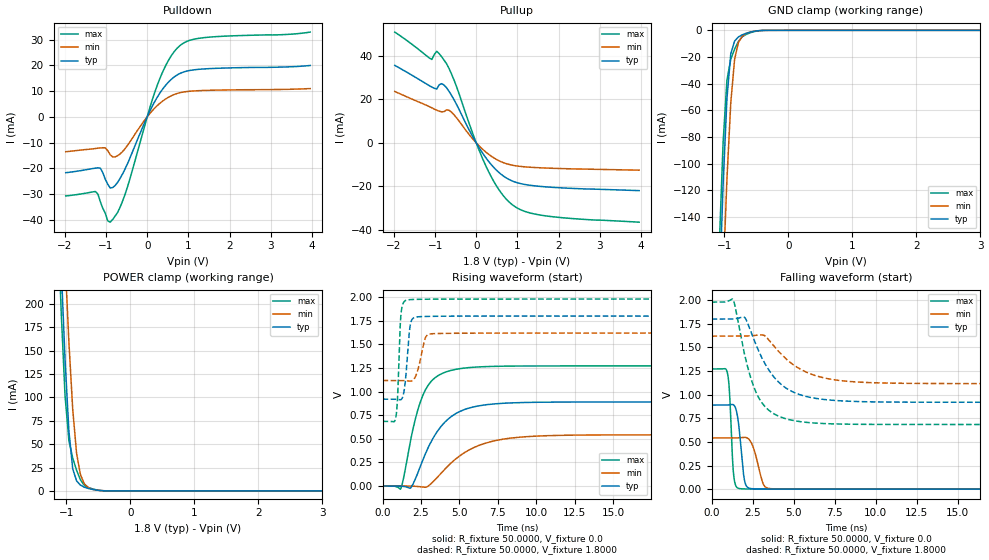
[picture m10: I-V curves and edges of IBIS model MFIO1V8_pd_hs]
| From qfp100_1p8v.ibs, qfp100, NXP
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[Model] MFIO1V8_pd_hs
|   Model MFIO1V8_pd_hs
| This model was characterised for following simulation conditions:
| External (pad) voltage:
|   - Typ: 1.8V,   - Min: 1.62V,   - Max: 1.98V
| Library cells for typ/min/max conditions are connected as defined below:
|  IO - External Pad
|  A - Core Input
|  EN - Output Buffer Enable
|  BOOST - vdde
|  EHS - vdd
|  ENZI - vdd
|  EPD - vdd
|  EPUN - vdd
|  ZI - NC
|  ZIF - NC
|  gnd - gnd
|  gnde - gnde
|  vdd - vdd
|  vdde - vdde
| All other pins connected to ground
Model_type I/O
Polarity   Non-Inverting
Enable   Active-Low
Vinl =   0.5400V
Vinh =   1.2600V
Vmeas =  0.9000V
Cref =   0.0F
Rref =   100.0000
Vref =   0.0V
C_comp   1.5958pF   1.5126pF   1.6704pF
|C_comp_pullup   0.7898pF   0.8219pF   0.7460pF
|C_comp_pulldown   0.5931pF   0.6315pF   0.5575pF
[Model Spec]
| variable   typ   min   max
Vinh   0.5400V   0.4860V   0.5940V
Vinl   1.2600V   1.1340V   1.3860V
Vmeas   0.9000V   0.8100V   0.9900V
[Temperature Range]   25.0000   0.1250k   -40.0000
[Voltage Range]   1.8000V   1.6200V   1.9800V
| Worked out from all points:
|   slope of the pulldown table from 0 to 0.27 V, typ, clamps not added: 32.6 ohm
|   slope of the pullup table from 0 to 0.27 V, typ, clamps not added: 34.8 ohm
|   GND clamp passes 1 mA (typ) near -0.56 V on its own axis
|   POWER clamp passes 1 mA (typ) near -0.54 V on its own axis
|   rising waveform, R_fixture 50.0000, V_fixture 0.0: 20-80 % time 1.9ns typ, 2.67ns min, 1.22ns max; typ from 0 V to 0.89 V
|   rising waveform, R_fixture 50.0000, V_fixture 1.8000: 20-80 % time 264ps typ, 419ps min, 177ps max; typ from 0.92 V to 1.8 V
|   falling waveform, R_fixture 50.0000, V_fixture 0.0: 20-80 % time 304ps typ, 487ps min, 201ps max; typ from 0.89 V to 0 V
|   falling waveform, R_fixture 50.0000, V_fixture 1.8000: 20-80 % time 1.84ns typ, 2.29ns min, 1.28ns max; typ from 1.8 V to 0.92 V
[Pulldown]
|Voltage   I(typ)   I(min)   I(max)
-1.98V    -21.74mA   -13.58mA   -30.76mA
-1.26V    -19.96mA   -12.33mA   -29.04mA
-1.14V    -19.96mA   -12.1mA    -33mA
-960mV    -26.19mA   -13.15mA   -40.44mA
-840mV    -27.51mA   -15.58mA   -39.92mA
-540mV    -20.34mA   -12.41mA   -30.2mA
60mV      2.086mA    1.197mA    3.341mA
300mV     9.043mA    5.145mA    14.58mA
540mV     13.88mA    7.813mA    22.59mA
840mV     17.16mA    9.517mA    28.23mA
1.44V     18.67mA    10.27mA    30.87mA
3.96V     19.95mA    10.98mA    32.93mA
[Pullup]
|Voltage   I(typ)   I(min)   I(max)
-1.98V    35.7mA     23.68mA    51.03mA
-1.08V    25.71mA    16.17mA    38.42mA
-960mV    24.81mA    15.04mA    42.18mA
-840mV    27.29mA    14.27mA    39.65mA
-720mV    25.36mA    15.21mA    36.42mA
-540mV    19.88mA    12.94mA    28.95mA
-60mV     2.001mA    1.263mA    3.041mA
240mV     -7.02mA    -4.333mA   -10.88mA
600mV     -14.41mA   -8.644mA   -22.88mA
900mV     -17.74mA   -10.36mA   -28.83mA
1.74V     -20.33mA   -11.62mA   -33.75mA
3.96V     -22mA      -12.58mA   -36.53mA
[GND_clamp]
|Voltage   I(typ)   I(min)   I(max)
-1.98V    -1.781A    -1.801A    -1.77A
-1.08V    -200.1mA   -270.2mA   -162.2mA
-1.02V    -116mA     -186.2mA   -84.49mA
-960mV    -51.26mA   -111.8mA   -37.36mA
-900mV    -17.65mA   -54.44mA   -21.7mA
-840mV    -8.02mA    -21.7mA    -14.08mA
-780mV    -4.924mA   -8.964mA   -8.313mA
-720mV    -3.338mA   -4.442mA   -4.753mA
-600mV    -1.403mA   -1.338mA   -1.896mA
-480mV    -330.4uA   -347.3uA   -423.3uA
-360mV    -26.82uA   -39.45uA   -30.02uA
3.96V     0A         0A         0A
[POWER_clamp]
|Voltage   I(typ)   I(min)   I(max)
-1.98V    2.119A     2.147A     2.105A
-1.14V    349.2mA    450mA      300.6mA
-1.08V    239.1mA    345.9mA    191.2mA
-1.02V    140.4mA    247.8mA    101.7mA
-960mV    64.08mA    159.3mA    53.89mA
-900mV    23.59mA    87.23mA    35.11mA
-840mV    10.79mA    40.2mA     22.07mA
-780mV    6.218mA    17.5mA     11.92mA
-720mV    4.013mA    7.752mA    6.009mA
-600mV    1.739mA    1.846mA    2.368mA
-360mV    67.5uA     96.07uA    73.34uA
3.96V     0A         0A         0A
[Ramp]
| variable   typ   min   max
dV/dt_r  0.5338/1.8998n   0.3252/2.6754n   0.7629/1.2220n
dV/dt_f  0.5279/1.8405n   0.3013/2.2918n   0.7771/1.2844n
R_load = 50.0000
[Rising Waveform]
R_fixture= 50.0000
V_fixture= 0.0
V_fixture_min= 0.0
V_fixture_max= 0.0
|time   V(typ)   V(min)   V(max)
0s        1.134nV    103.8nV    53.92pV
1.185ns   -399.3uV   61.24uV    -28.51mV
1.826ns   -20.58mV   -118.7uV   484.5mV
2.193ns   96.8mV     -3.408mV   747mV
3.08ns    443.4mV    14.29mV    1.092V
4.209ns   701.1mV    204mV      1.213V
5.822ns   833.9mV    397.5mV    1.257V
8.271ns   879.5mV    505.9mV    1.27V
12.75ns   889.3mV    539.3mV    1.272V
100ns     889.7mV    541.9mV    1.272V
[Rising Waveform]
R_fixture= 50.0000
V_fixture= 1.8000
V_fixture_min= 1.6200
V_fixture_max= 1.9800
|time   V(typ)   V(min)   V(max)
0s        919.5mV    1.117V     684.3mV
854ps     919.6mV    1.117V     718.6mV
973.1ps   917.2mV    1.117V     922.4mV
1.219ns   917mV      1.118V     1.847V
1.468ns   1.086V     1.115V     1.962V
1.755ns   1.649V     1.11V      1.973V
2.224ns   1.79V      1.192V     1.976V
2.823ns   1.796V     1.581V     1.978V
3.436ns   1.797V     1.614V     1.978V
100ns     1.799V     1.619V     1.979V
[Falling Waveform]
R_fixture= 50.0000
V_fixture= 0.0
V_fixture_min= 0.0
V_fixture_max= 0.0
|time   V(typ)   V(min)   V(max)
0s        889.7mV    541.9mV    1.272V
965.7ps   890.1mV    542mV      1.23V
1.095ns   892.5mV    541.9mV    1.018V
1.36ns    888.9mV    541.7mV    127.4mV
1.585ns   766.4mV    542.9mV    13.03mV
1.819ns   387.9mV    546.5mV    3.965mV
2.158ns   25.18mV    543mV      1.973mV
3.176ns   1.574mV    46.27mV    615.5uV
3.853ns   843.4uV    2.965mV    324.8uV
100ns     11.12nV    119.5nV    6.01nV
[Falling Waveform]
R_fixture= 50.0000
V_fixture= 1.8000
V_fixture_min= 1.6200
V_fixture_max= 1.9800
|time   V(typ)   V(min)   V(max)
0s        1.799V     1.619V     1.979V
1.326ns   1.8V       1.619V     2.003V
1.987ns   1.82V      1.619V     1.445V
2.301ns   1.71V      1.622V     1.228V
2.693ns   1.535V     1.627V     1.031V
3.173ns   1.354V     1.629V     889.9mV
4.415ns   1.084V     1.398V     750.9mV
6.093ns   968.4mV    1.216V     701.7mV
13.05ns   919.8mV    1.118V     684.2mV
100ns     919.5mV    1.117V     684.3mV
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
